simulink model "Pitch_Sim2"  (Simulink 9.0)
settings: Solver=ode45  StartTime=0.0  StopTime=100  RelTol=1e-3  EnableMultiTasking=on
InitFcn:
  | init_pitch;
StopFcn:
  | pl
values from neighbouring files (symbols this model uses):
  Cza = -0.032    [init_pitch.m]    (also in init.m)
  Czde = -0.0087    [init_pitch.m]    (also in init.m)
  d2r = pi/180    (= 0.0174532925199)    [frequ.m]    (also in init_pitch.m; pl.m; init.m; freq.m)
  Mv = 1219.1    [init_pitch.m]    (also in init.m; init_lat.m)
  Qbar = 1220.6    [init_pitch.m]    (also in init.m; init_lat.m)
  r2d = 180/pi    (= 57.2957795131)    [frequ.m]    (also in init_pitch.m; pl.m; init.m; freq.m)
  Sref = 145.4    [init_pitch.m]    (also in init.m; init_lat.m)
undefined symbols (not defined in the file or in its folder): Ap, Bp, Cp, Dp, Kc

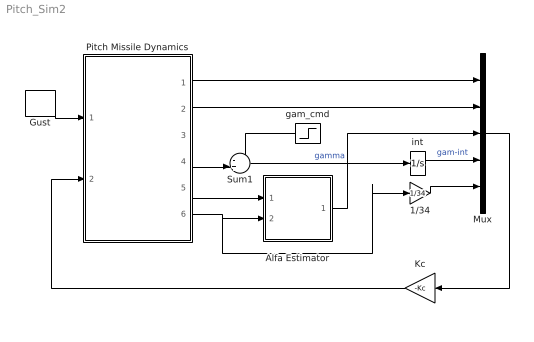
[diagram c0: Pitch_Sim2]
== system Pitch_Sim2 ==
  1/34 : Gain  Gain=1/34
  Alfa Estimator : Subsystem
  Gust : DiscretePulseGenerator  PulseType=Time based  Amplitude=30  Period=200  PulseWidth=2  PhaseDelay=10
  Kc : Gain  Gain=-Kc  Multiplication=Matrix(K*u)
  Mux : Mux  Inputs=5
  Pitch Missile Dynamics : Subsystem
  Sum1 : Sum  Inputs=-+|
  gam_cmd : Step  Time=0  After=1*d2r  SampleTime=0
  int : Integrator
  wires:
  Mux/1 -> Kc/1
  Pitch Missile Dynamics/1(theta) -> Mux/1
  Pitch Missile Dynamics/2(q) -> Mux/2
  Pitch Missile Dynamics/4(gama) -> Sum1/2
  int/1 -> Mux/4  "gam-int"
  Sum1/1 -> int/1  "gamma"
  Kc/1 -> Pitch Missile Dynamics/2(Elevon)
  1/34/1 -> Mux/5
  Pitch Missile Dynamics/5(Nz) -> Alfa Estimator/1(Nz)
  Pitch Missile Dynamics/6(delevn) -> 1/34/1, Alfa Estimator/2(d-elev)
  Alfa Estimator/1(alf_est) -> Mux/3
  Gust/1 -> Pitch Missile Dynamics/1(WGust)
  gam_cmd/1 -> Sum1/1

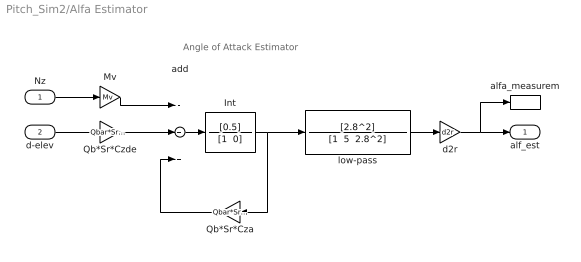
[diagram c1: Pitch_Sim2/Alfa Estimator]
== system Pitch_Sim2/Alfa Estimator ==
  note: Angle of Attack Estimator
  Nz : Inport
  d-elev : Inport  Port=2
  Int : TransferFcn  Numerator=[0.5]  Denominator="[1  0]"
  Mv : Gain  Gain=Mv
  Qb*Sr*Cza : Gain  Gain=Qbar*Sref*Cza
  Qb*Sr*Czde : Gain  Gain=Qbar*Sref*Czde*r2d
  add : Sum  Inputs=-++
  alfa_measurem : ToWorkspace  VariableName=alfest  SampleTime=-1
  d2r : Gain  Gain=d2r
  low-pass : TransferFcn  Numerator=[2.8^2]  Denominator="[1  5  2.8^2]"
  alf_est : Outport
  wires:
  d2r/1 -> alfa_measurem/1, alf_est/1
  low-pass/1 -> d2r/1
  Nz/1 -> Mv/1
  d-elev/1 -> Qb*Sr*Czde/1
  Int/1 -> low-pass/1, Qb*Sr*Cza/1
  Qb*Sr*Czde/1 -> add/2
  Mv/1 -> add/1
  Qb*Sr*Cza/1 -> add/3
  add/1 -> Int/1

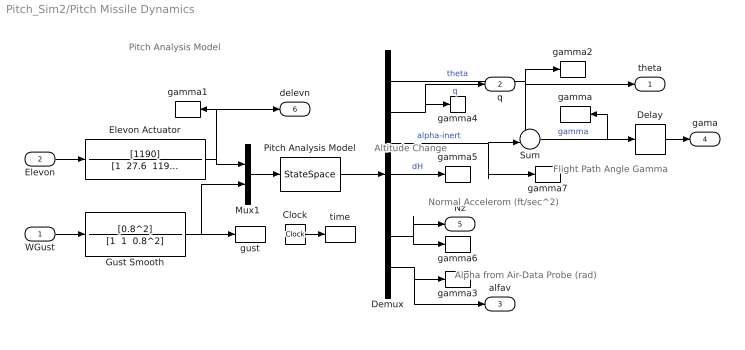
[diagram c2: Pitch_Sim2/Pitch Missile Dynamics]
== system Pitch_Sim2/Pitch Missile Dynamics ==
  note: Pitch Analysis Model
  note: Flight Path Angle Gamma
  note: Alpha from Air-Data Probe (rad)
  note: Normal Accelerom (ft/sec^2)
  note: Altitude Change
  WGust : Inport
  Elevon : Inport  Port=2
  Clock : Clock
  Delay : TransportDelay  DelayTime=0.7  PadeOrder=2
  Demux : Demux  Outputs=7
  Elevon Actuator : TransferFcn  Numerator=[1190]  Denominator="[1  27.6  1190]"
  Gust Smooth : TransferFcn  Numerator=[0.8^2]  Denominator="[1  1  0.8^2]"
  Mux1 : Mux  Inputs=2
  Pitch Analysis Model : StateSpace  A=Ap  B=Bp  C=Cp  D=Dp  InitialCondition=0
  Sum : Sum  Inputs=+-|
  gamma : ToWorkspace  VariableName=Gam  SampleTime=-1
  gamma1 : ToWorkspace  VariableName=Elev  SampleTime=-1
  gamma2 : ToWorkspace  VariableName=Thet  SampleTime=-1
  gamma3 : ToWorkspace  VariableName=alfav  SampleTime=-1
  gamma4 : ToWorkspace  VariableName=q  SampleTime=-1
  gamma5 : ToWorkspace  VariableName=altit  SampleTime=-1
  gamma6 : ToWorkspace  VariableName=Az  SampleTime=-1
  gamma7 : ToWorkspace  VariableName=alfin  SampleTime=-1
  gust : ToWorkspace  VariableName=gust  SampleTime=-1
  time : ToWorkspace  VariableName=time  SampleTime=-1
  theta : Outport
  q : Outport  Port=2
  alfav : Outport  Port=3
  gama : Outport  Port=4
  Nz : Outport  Port=5
  delevn : Outport  Port=6
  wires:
  Demux/1 -> theta/1, Sum/1, gamma2/1  "theta"
  Delay/1 -> gama/1
  Pitch Analysis Model/1 -> Demux/1
  Demux/3 -> gamma7/1, Sum/2  "alpha-inert"
  Demux/2 -> q/1, gamma4/1  "q"
  Clock/1 -> time/1
  Demux/4 -> gamma5/1  "dH"
  Demux/6 -> Nz/1, gamma6/1
  Sum/1 -> gamma/1, Delay/1  "gamma"
  Gust Smooth/1 -> gust/1, Mux1/2
  WGust/1 -> Gust Smooth/1
  Mux1/1 -> Pitch Analysis Model/1
  Demux/7 -> alfav/1, gamma3/1
  Elevon/1 -> Elevon Actuator/1
  Elevon Actuator/1 -> delevn/1, gamma1/1, Mux1/1
